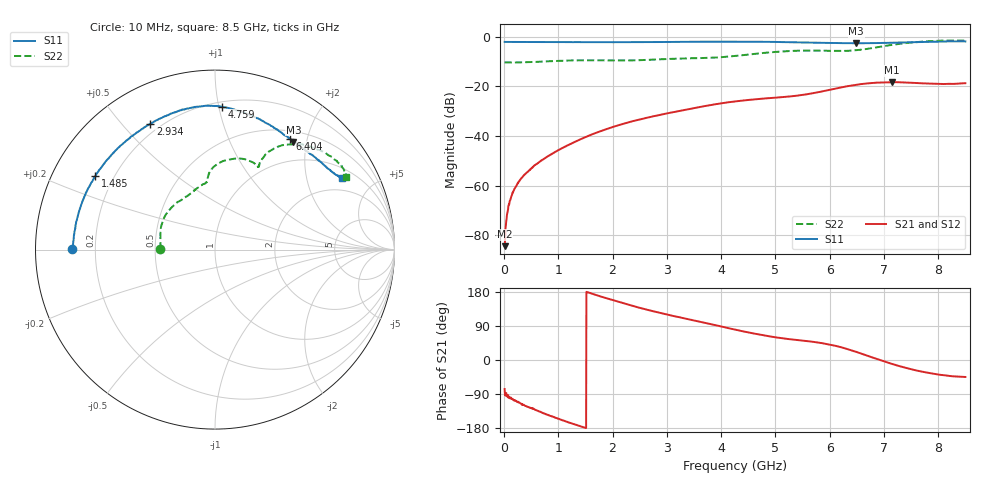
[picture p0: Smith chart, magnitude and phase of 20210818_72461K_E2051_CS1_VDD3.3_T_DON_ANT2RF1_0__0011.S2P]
!Agilent Technologies,E5071C,MY46417908,A.11.23
!Date: Wed Aug 18 14:24:27 2021
!Data & Calibration Information:
!Freq	S11:SOLT2(ON)	S21:SOLT2(ON)	S12:SOLT2(ON)	S22:SOLT2(ON)
!PortZ  Port1:50+j0  Port2:50+j0
!Above PortZ is port z conversion or system Z0 setting when saving the data.
!When reading, reference impedance value at option line is always used.
# Hz S dB R 50
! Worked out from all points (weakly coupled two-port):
!   1601 points, 10 MHz to 8.5 GHz, reference 50 ohm
!   highest |S21| = -18.26 dB at 7.152 GHz (marker M1); lowest = -84.4 dB at 10 MHz (marker M2)
!   lowest |S11| = -2.6 dB at 6.489 GHz (marker M3), VSWR 6.77, Z = 33.1 + j88.7 ohm
!   |S11| at or under -10 dB: nowhere
!   |S22| runs from -10.3 to -1.4 dB; largest |S21 - S12| = 0.00053
!   S11 on the Smith chart (normalised r, x): 10 MHz: 0.11, +0.00; 1.485 GHz: 0.13, +0.28; 2.934 GHz: 0.16, +0.60; 4.759 GHz: 0.23, +1.02; 6.404 GHz: 0.62, +1.72; 8.5 GHz: 1.41, +3.25
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1e7  -2.00 179.7  -84.44 -76.7  -88.41 -82.5  -10.27 179.6
3.653125e7  -2.03 179.2  -75.30 -87.4  -76.45 -87.7  -10.30 179.1
8.42875e7  -2.03 178.2  -67.97 -97.0  -67.88 -94.9  -10.31 178.0
1.267375e8  -2.03 177.3  -64.98 -101.6  -64.61 -101.6  -10.32 176.9
2.116375e8  -2.06 175.5  -60.58 -107.8  -60.50 -108.4  -10.32 174.8
3.28375e8  -2.06 173.1  -56.84 -116.3  -56.78 -116.2  -10.26 172.5
7.10425e8  -2.08 164.9  -49.56 -139.7  -49.57 -139.5  -9.97 163.1
1.426769e9  -2.12 149.8  -41.13 -175.8  -41.11 -176.0  -9.46 141.6
1.485138e9  -2.13 148.5  -40.56 -178.7  -40.55 -178.8  -9.45 139.7
2.127194e9  -2.14 134.4  -35.52 152.7  -35.52 152.6  -9.52 122.0
2.843538e9  -2.08 119.0  -31.61 125.3  -31.61 125.3  -9.08 108.3
2.933744e9  -2.07 117.2  -31.20 122.5  -31.19 122.5  -9.00 106.8
4.255e9  -1.91 94.4  -26.05 80.3  -26.05 80.2  -7.71 95.3
4.759094e9  -1.97 87.2  -24.92 65.7  -24.92 65.8  -6.52 89.2
5.671769e9  -2.30 71.2  -22.80 48.4  -22.81 48.5  -5.52 68.7
6.404031e9  -2.55 55.8  -19.62 25.4  -19.63 25.3  -5.52 62.3
6.488931e9  -2.59 53.9  -19.35 21.4  -19.37 21.3  -5.40 62.6
7.088538e9  -2.39 42.4  -18.29 -7.7  -18.32 -7.8  -3.41 58.4
7.152212e9  -2.37 41.3  -18.26 -10.5  -18.29 -10.5  -3.20 57.3
7.497119e9  -2.23 35.7  -18.50 -24.2  -18.50 -24.3  -2.31 49.6
7.942844e9  -1.94 31.0  -18.93 -37.0  -18.92 -37.0  -1.61 38.1
8.5e9  -1.84 29.4  -18.69 -44.8  -18.70 -45.0  -1.57 28.9
